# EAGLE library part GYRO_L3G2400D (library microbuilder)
L3G4200D - 3-Axis MEMS gyroscope/motion sensor Three selectable scales: 250/500/2000 dps 1²C/SPI Interface 16-bit data 8-bit temperature VDD: 2.4-3.6V (IO 1.8V compatible) -40°C-85°C
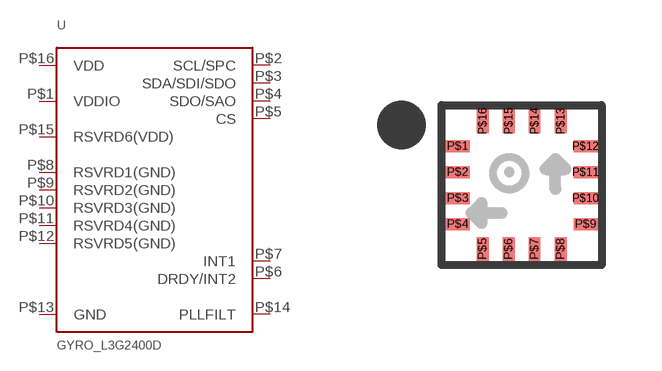
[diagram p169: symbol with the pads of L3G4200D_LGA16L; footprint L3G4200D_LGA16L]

Designator prefix U

## GYRO_L3G2400D  [L3G4200D_LGA16L]
P$1  VDDIO  pwr
P$2  SCL/SPC
P$3  SDA/SDI/SDO
P$4  SDO/SAO
P$5  CS
P$6  DRDY/INT2
P$7  INT1
P$8  RSVRD1(GND)
P$9  RSVRD2(GND)
P$10  RSVRD3(GND)
P$11  RSVRD4(GND)
P$12  RSVRD5(GND)
P$13  GND
P$14  PLLFILT
P$15  RSVRD6(VDD)
P$16  VDD

## Footprint L3G4200D_LGA16L (pad centres in mm)
smd 0.6 x 0.3: P$1 -1.6,0.975; P$2 -1.6,0.325; P$3 -1.6,-0.325; P$4 -1.6,-0.975; P$9 1.6,-0.975; P$10 1.6,-0.325; P$11 1.6,0.325; P$12 1.6,0.975
smd 0.3 x 0.6: P$5 -0.975,-1.6; P$6 -0.325,-1.6; P$7 0.325,-1.6; P$8 0.975,-1.6; P$13 0.975,1.6; P$14 0.325,1.6; P$15 -0.325,1.6; P$16 -0.975,1.6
